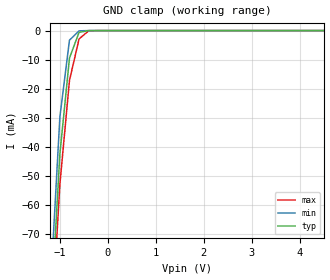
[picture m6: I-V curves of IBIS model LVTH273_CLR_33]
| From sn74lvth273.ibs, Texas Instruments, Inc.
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|   Model LVTH273_CLR_33
[Model]   LVTH273_CLR_33
Model_type  Input
Polarity   Non-Inverting
Vinl = 0.8V
Vinh = 2.0V
| variable   typ   min   max
C_comp   4pf   NA   NA
[Temperature Range]   40   -25   100
| Ambient temperature   25   -40   85
[Voltage range]   3.3   3.0   3.6
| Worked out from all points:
|   GND clamp passes 1 mA (typ) near -0.61 V on its own axis
[GND Clamp]
|   Voltage   I(typ)   I(min)   I(max)
-5V       -1.926A    -2.125A    -1.756A
-1.2V     -101.7mA   -90.21mA   -110.2mA
-1V       -42.55mA   -29.79mA   -53.03mA
-800mV    -9.474mA   -3.309mA   -17.2mA
-600mV    -627.3uA   -92.07uA   -2.88mA
-400mV    -2.645uA   -67.63nA   -92.25uA
5V        100.5pA    6.52pA     272.5pA
